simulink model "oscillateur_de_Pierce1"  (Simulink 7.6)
settings: Solver=ode15s  StartTime=0.0  StopTime=0.1  RelTol=1e-3
libraries: fl_lib x6, nesl_utility x2, elec_lib x1

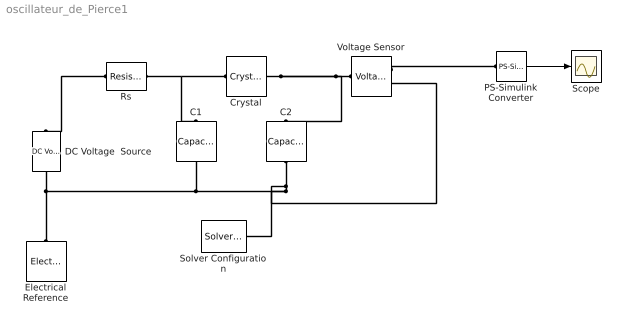
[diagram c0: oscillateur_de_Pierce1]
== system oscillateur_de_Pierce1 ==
  C1 : fl_lib/Electrical/Electrical Elements/Capacitor  DialogController=NetworkEngine.DynNeDlgSource  SystemSampleTime=-1  c=0.1 pF  v0=0 V  r=1e-22 Ohm  g=0 1/Ohm  i_Log=off  v_Log=off  vc_Log=off  LocalVarNames=|i|v|vc  LocalVarDescs=|i|v|Internal variable for voltage across capacitor term  LocalVarLogging=[0 0 0]
  C2 : fl_lib/Electrical/Electrical Elements/Capacitor  DialogController=NetworkEngine.DynNeDlgSource  SystemSampleTime=-1  c=0.1 pF  v0=0 V  r=1e-22 Ohm  g=0 1/Ohm  i_Log=off  v_Log=off  vc_Log=off  LocalVarNames=|i|v|vc  LocalVarDescs=|i|v|Internal variable for voltage across capacitor term  LocalVarLogging=[0 0 0]
  Crystal : elec_lib/Passive Devices/Crystal  DialogController=NetworkEngine.DynNeDlgSource  SystemSampleTime=-1  param=1  L1=6.742e+3 H  Fs=32.764 kHz  Fa=32.768 kHz  param_R1=1  R1=15 kOhm  Q=9e+4  C1=0.0035 pF  CL=12.5 pF  C0=1.6 pF  V_ini=0 V  LocalVarLogging=[]
  DC Voltage  Source : fl_lib/Electrical/Electrical Sources/DC Voltage Source  DialogController=NetworkEngine.DynNeDlgSource  SystemSampleTime=-1  v0=1.4 V  i_Log=off  v_Log=off  LocalVarNames=|i|v  LocalVarDescs=|i|v  LocalVarLogging=[0 0]
  Electrical Reference : fl_lib/Electrical/Electrical Elements/Electrical Reference  DialogController=NetworkEngine.DynNeDlgSource  SystemSampleTime=-1  i_Log=off  LocalVarNames=|i  LocalVarDescs=|i  LocalVarLogging=0
  PS-Simulink Converter : nesl_utility/PS-Simulink Converter  DialogController=NetworkEngine.DynNeUtilDlgSource  SystemSampleTime=-1  PhysicalDomain=network_engine_domain  LeftPortType=input  RightPortType=output  SubClassName=ps_output  Unit=1  AffineConversion=off
  Rs : fl_lib/Electrical/Electrical Elements/Resistor  DialogController=NetworkEngine.DynNeDlgSource  SystemSampleTime=-1  R=10 kOhm  i_Log=off  v_Log=off  LocalVarNames=|i|v  LocalVarDescs=|i|v  LocalVarLogging=[0 0]
  Scope : Scope
  Solver Configuration : nesl_utility/Solver Configuration  DialogController=NetworkEngine.DynNeUtilDlgSource  SystemSampleTime=-1  PhysicalDomain=network_engine_domain  LeftPortType=input  RightPortType=generic  SubClassName=solver  Accelerate=off  Profile=off  ResidualTolerance=1e-9  MaxNonlinIter=3  MaxModeIter=2  DoFixedCost=off  UseLocalSampling=off  DoDC=off  LinearAlgebra=Sparse  LocalSolverSampleTime=.001  LocalSolverChoice=NE_BACKWARD_EULER_ADVANCER  UseLocalSolver=off
  Voltage Sensor : fl_lib/Electrical/Electrical Sensors/Voltage Sensor  DialogController=NetworkEngine.DynNeDlgSource  SystemSampleTime=-1  i1_Log=off  v1_Log=off  LocalVarNames=|i1|v1  LocalVarDescs=|i1|v1  LocalVarLogging=[0 0]
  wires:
  PS-Simulink Converter/1 -> Scope/1
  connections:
  Rs/LConn1 -- DC Voltage  Source/LConn1
  C2/RConn1 -- Solver Configuration/RConn1 -- C1/RConn1 -- DC Voltage  Source/RConn1 -- Electrical Reference/LConn1 -- Voltage Sensor/RConn2
  Rs/RConn1 -- Crystal/LConn1 -- C1/LConn1
  Voltage Sensor/LConn1 -- Crystal/RConn1 -- C2/LConn1
  Voltage Sensor/RConn1 -- PS-Simulink Converter/LConn1
